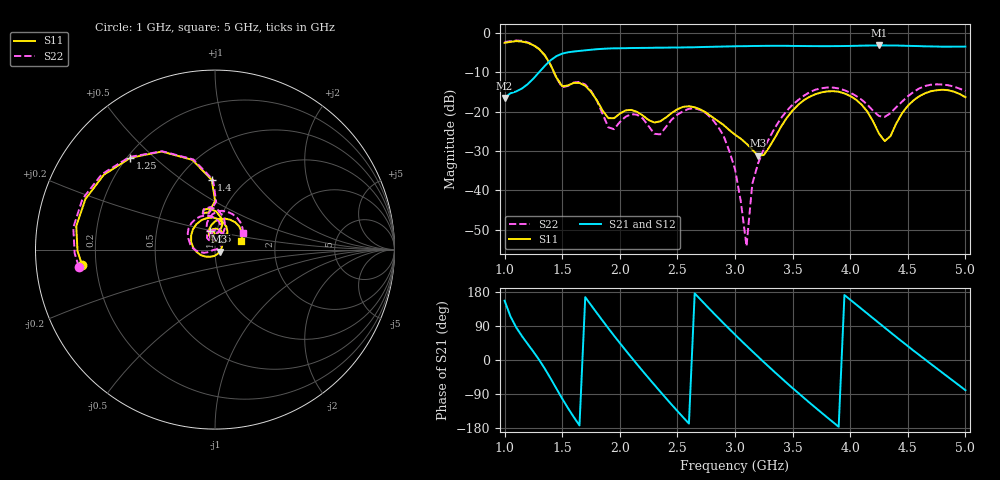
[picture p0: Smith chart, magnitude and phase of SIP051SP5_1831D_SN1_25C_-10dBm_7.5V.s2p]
# GHz  S  dB  R  50
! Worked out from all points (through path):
!   81 points, 1 GHz to 5 GHz, reference 50 ohm
!   highest |S21| = -3.20 dB at 4.25 GHz (marker M1); lowest = -16.6 dB at 1 GHz (marker M2)
!   lowest |S11| = -31.2 dB at 3.2 GHz (marker M3), VSWR 1.06, Z = 52.6 - j1.15 ohm
!   |S11| at or under -10 dB: 1.429 GHz to end of sweep
!   |S22| runs from -54.1 to -1.9 dB; largest |S21 - S12| = 0.0036
!   S11 on the Smith chart (normalised r, x): 1 GHz: 0.15, -0.05; 1.25 GHz: 0.21, +0.42; 1.4 GHz: 0.71, +0.65; 2.5 GHz: 0.93, +0.20; 5 GHz: 1.33, +0.13
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1  -2.54 -173.6  -16.57 156.6  -16.54 156.5  -2.33 -172.9
1.25  -3.16 132.6  -11.62 21.9  -11.60 21.8  -3.07 132.7
1.4  -8.20 92.7  -6.96 -49.0  -6.95 -48.9  -8.20 91.6
1.55  -13.36 108.6  -4.95 -126.9  -4.93 -126.9  -13.48 108.8
1.7  -13.44 88.0  -4.45 165.9  -4.45 165.9  -13.15 85.3
1.9  -21.65 87.1  -4.00 83.9  -4.00 83.9  -23.97 76.9
2.1  -19.56 99.1  -3.87 7.1  -3.86 7.1  -20.64 100.2
2.35  -22.48 107.3  -3.79 -83.1  -3.79 -83.2  -25.77 113.3
2.5  -19.41 103.9  -3.75 -134.7  -3.74 -134.6  -20.76 118.4
2.7  -19.44 69.5  -3.62 159.8  -3.62 159.8  -19.61 77.5
2.85  -22.34 49.5  -3.53 112.6  -3.52 112.7  -23.71 47.0
3  -25.85 35.9  -3.42 67.1  -3.42 67.1  -34.58 23.4
3.1  -28.14 18.1  -3.39 37.6  -3.38 37.5  -54.13 -168.0
3.15  -29.64 2.2  -3.35 23.1  -3.36 23.1  -38.35 -166.3
3.2  -31.17 -23.2  -3.34 8.7  -3.34 8.7  -33.16 -162.6
3.45  -21.57 -158.1  -3.31 -60.7  -3.31 -60.7  -19.77 -175.8
3.7  -15.56 137.6  -3.39 -126.2  -3.39 -126.1  -14.42 140.6
3.95  -15.38 82.9  -3.36 171.4  -3.36 171.3  -14.57 97.0
4.25  -25.58 52.8  -3.20 97.5  -3.21 97.6  -21.12 86.4
4.35  -26.20 101.6  -3.23 73.0  -3.23 73.1  -20.41 106.7
4.65  -15.35 81.2  -3.44 1.3  -3.43 1.4  -13.50 87.5
5  -16.35 17.5  -3.50 -79.7  -3.50 -79.6  -14.80 30.6
